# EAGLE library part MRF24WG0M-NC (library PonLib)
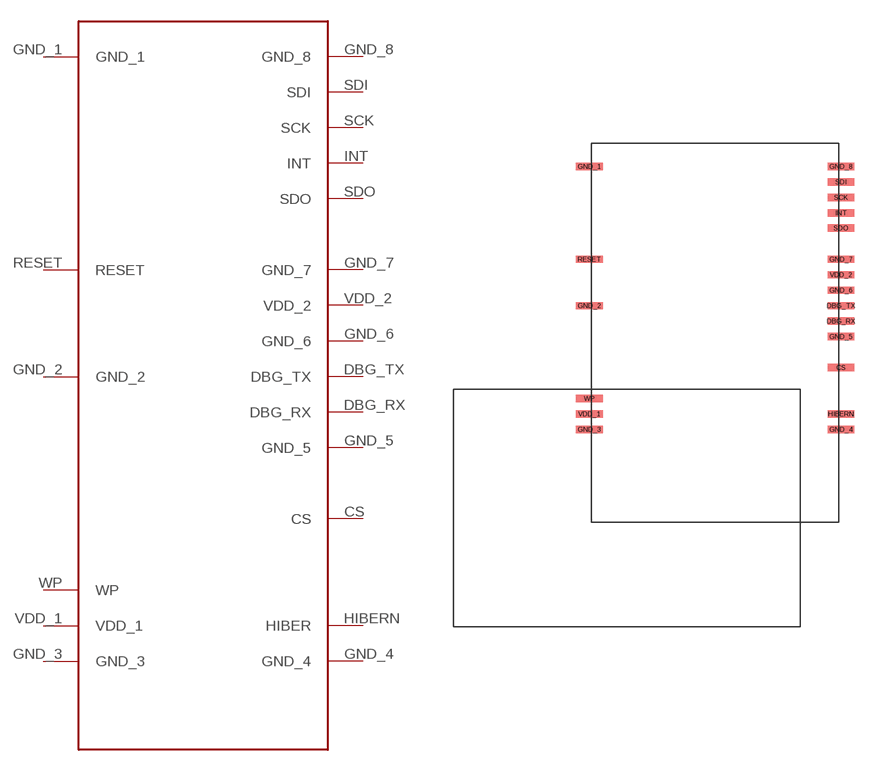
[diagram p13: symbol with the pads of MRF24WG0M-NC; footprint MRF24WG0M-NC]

Designator prefix -

## MRF24WG0M-NC  [MRF24WG0M-NC]
CS  CS
DBG_RX  DBG_RX
DBG_TX  DBG_TX
GND_1  GND_1
GND_2  GND_2
GND_3  GND_3
GND_4  GND_4
GND_5  GND_5
GND_6  GND_6
GND_7  GND_7
GND_8  GND_8
HIBERN  HIBER
INT  INT
RESET  RESET
SCK  SCK
SDI  SDI
SDO  SDO
VDD_1  VDD_1
VDD_2  VDD_2
WP  WP

## Footprint MRF24WG0M-NC (pad centres in mm)
smd 2.2 x 0.6: CS 10.338,-5.715; DBG_RX 10.338,-1.905; DBG_TX 10.338,-0.635; GND_1 -10.338,10.795; GND_2 -10.338,-0.635; GND_3 -10.338,-10.795; GND_4 10.338,-10.795; GND_5 10.338,-3.175; GND_6 10.338,0.635; GND_7 10.338,3.175; GND_8 10.338,10.795; HIBERN 10.338,-9.525; INT 10.338,6.985; RESET -10.338,3.175; SCK 10.338,8.255; SDI 10.338,9.525; SDO 10.338,5.74; VDD_1 -10.338,-9.525; VDD_2 10.338,1.905; WP -10.338,-8.255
